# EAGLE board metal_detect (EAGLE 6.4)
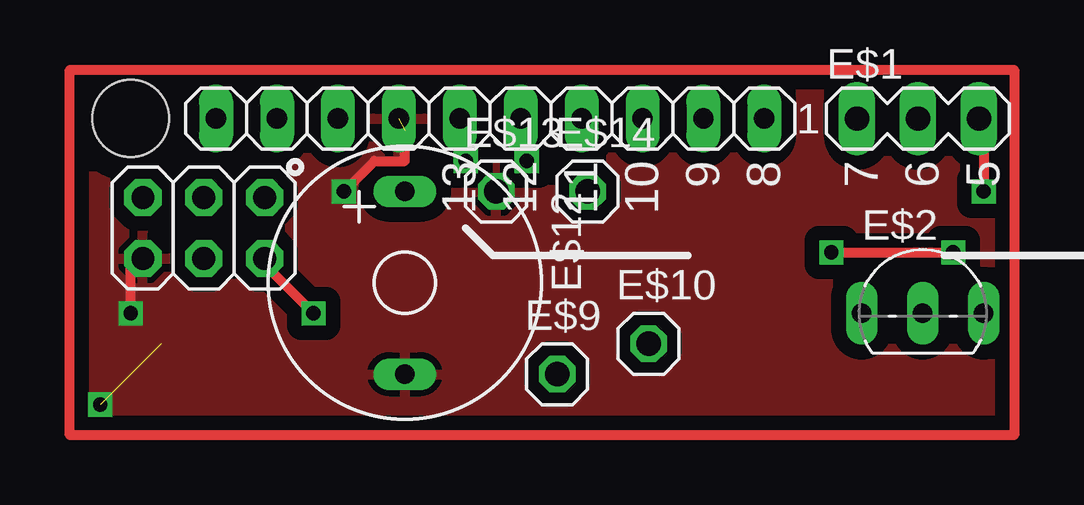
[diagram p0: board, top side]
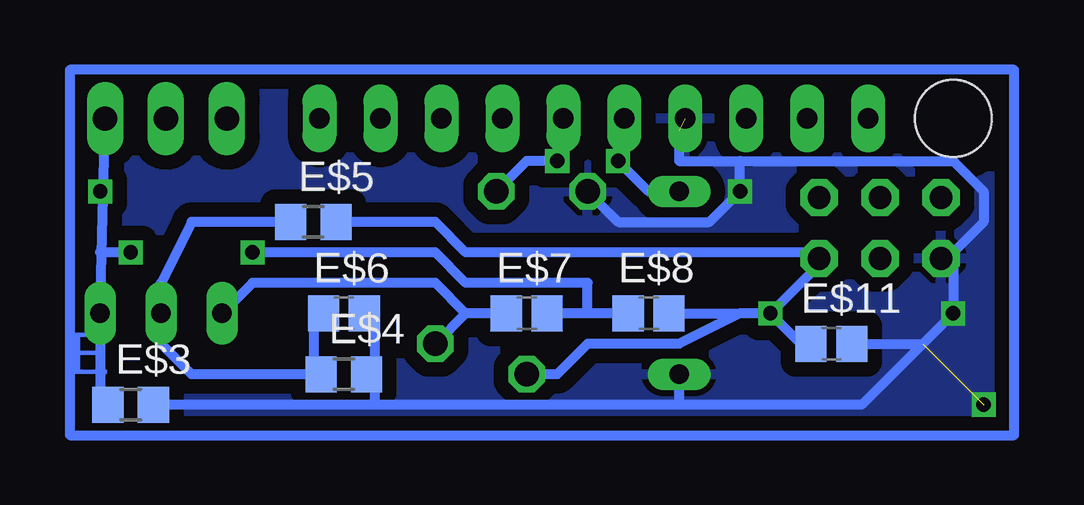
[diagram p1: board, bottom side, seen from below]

No outline drawn. Coordinates in mm, seen from the top.
Copper layers (1*16): Top 0.035mm / dielectric 1.5mm / Bottom 0.035mm
Design rules "default *": minimum track width 10mil, minimum drill 24mil, track to track 24mil, track to pad 24mil, pad to pad 24mil, via to via 24mil, smd to smd 24mil, copper to edge 40mil, drill to drill 8mil, minimum pad ring 10mil, minimum via ring 8mil, stop-mask expansion 4mil, vias tented up to drill 0mil, thermal gap 10mil
Net classes: 0 default: width 0.254 mm, clearance 0.254 mm; 2 gnd: width 0.305 mm, drill 0.559 mm, clearance 0.254 mm; 3 usbvcc: width 0.508 mm, drill 0.61 mm, clearance 0.254 mm; 4 aref: width 0.406 mm, drill 0.61 mm, clearance 0.254 mm
Holes 3.2 mm at 2.54,13.21

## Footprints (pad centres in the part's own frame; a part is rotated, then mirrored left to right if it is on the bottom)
MA03-1 = drill 1.016 long: 1 -2.54,0; 2 0,0; 3 2.54,0
TO92-BCE = drill 0.813 long: B 2.54,0; C 0,0; E -2.54,0
R0805 = smd 1.3 x 1.5: 1 -0.95,0; 2 0.95,0
C2012 = smd 1.3 x 1.5: 1 -0.85,0; 2 0.85,0
1X01 = drill 1.016 octagon: 1 0,0
BEEPER = drill 0.813 long: 1 -3.81,0; 2 3.81,0
2X03 = drill 0.95 pad 1.55 octagon: 1 -2.54,-1.27; 2 -2.54,1.27; 3 0,-1.27; 4 0,1.27; 5 2.54,-1.27; 6 2.54,1.27
1X10@1 = drill 0.85 pad 1.422 long: 1 -11.43,0; 2 -8.89,0; 3 -6.35,0; 4 -3.81,0; 5 -1.27,0; 6 1.27,0; 7 3.81,0; 8 6.35,0; 9 8.89,0; 10 11.43,0

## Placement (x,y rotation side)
E$1  [MA03-1]  35.36,13.2 0 top
E$2  [TO92-BCE]  35.56,5.08 0 top
E$3  1,2k  [R0805]  36.83,1.27 0 bottom
E$4  10k  [R0805]  27.94,2.54 0 bottom
E$5  1k  [R0805]  29.21,8.89 0 bottom
E$6  100n  [C2012]  27.94,5.08 0 bottom
E$7  22n  [C2012]  20.32,5.08 0 bottom
E$8  22n  [C2012]  15.24,5.08 0 bottom
E$9  [1X01]  20.32,2.54 0 top
E$10  [1X01]  24.13,3.81 0 top
E$11  100n  [C2012]  7.62,3.81 0 bottom
E$12  [BEEPER]  13.97,6.35 270 top
E$13  [1X01]  17.78,10.16 0 top
E$14  [1X01]  21.59,10.16 0 top
ICSP1  3x2 M  [2X03]  5.59,8.64 180 top
IOH  10x1F-H8.5  [1X10@1]  17.53,13.21 180 top

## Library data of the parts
E$1 = con-lstb
E$2 = transistor-npn
E$3-E$8 E$11 = rcl
E$9 E$10 E$13 E$14 = pinhead
E$12 = special
ICSP1 IOH = SmartPrj

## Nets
+5V [usbvcc]: ICSP1.2
AD4/SDA: IOH.9
AD5/SCL: IOH.10
AREF [aref]: IOH.8
GND [gnd]: E$12.2 E$13.1 ICSP1.6 IOH.7
IO8: IOH.1
IO9: IOH.2
MISO: IOH.5
MISO2: ICSP1.1
MOSI: IOH.4
MOSI2: ICSP1.4
RESET2: ICSP1.5
S$2: E$1.3 E$2.B
S$3: E$2.C
S$4: E$9.1
S$7: E$2.E
S$8: E$12.1
S$10: E$14.1
SCK: IOH.6
SCK2: ICSP1.3
SS: IOH.3

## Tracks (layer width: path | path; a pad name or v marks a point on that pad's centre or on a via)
GND  (via drill 0.6)  (2 unrouted)
  Top 0.406: v11.43,10.16 12.7,11.43 13.97,11.43 13.97,12.7 | v2.54,5.08 2.54,7.62
  Bottom 0.406: 26.67,1.27 35.56,1.27 | 3.81,3.81 v2.54,5.08 2.54,7.62 1.27,8.89 1.27,10.16 2.54,11.43 11.43,11.43 | 3.81,3.81 6.35,1.27 13.97,1.27 | 13.97,1.27 26.67,1.27 | 13.97,12.7 13.97,11.43 11.43,11.43 | 26.67,5.08 26.67,1.27 | 6.35,3.81 3.81,3.81 | E$12.2 13.97,1.27 | E$13.1 16.51,8.89 12.7,8.89 v11.43,10.16 11.43,11.43
  other vias: 1.27,1.27
  pour Bottom: 0,0 0,15.24 39.37,15.24 39.37,0
  pour Top: 0,0 0,15.24 39.37,15.24 39.37,0
S$1
  Bottom 0.406: 0,0 0,15.24 39.37,15.24 39.37,0 0,0
S$2
  Bottom 0.406: 38.1,1.27 E$2.B E$1.3
S$3
  Bottom 0.406: E$2.C 35.56,3.81 34.29,2.54 29.21,2.54 29.21,5.08
S$4  (via drill 0.6)
  Top 0.406: v10.16,5.08 7.62,7.62
  Bottom 0.406: 27.94,8.89 24.13,8.89 22.86,7.62 7.62,7.62 v10.16,5.08 | 13.97,5.08 11.43,5.08 | v10.16,5.08 11.43,5.08 | 8.89,3.81 v10.16,5.08 | 11.43,5.08 13.97,3.81 17.78,3.81 19.05,2.54 E$9.1
S$5
  Bottom 0.406: 30.48,8.89 34.29,8.89 35.56,6.35
S$6  (via drill 0.6)
  Top 0.406: v31.75,7.62 v36.83,7.62
  Bottom 0.406: 16.51,5.08 17.78,5.08 | 17.78,5.08 19.05,5.08 | 17.78,5.08 17.78,6.35 22.86,6.35 24.13,7.62 v31.75,7.62 | v36.83,7.62 38.1,7.62
S$7
  Bottom 0.406: 21.59,5.08 22.86,5.08 | 22.86,5.08 24.13,6.35 31.75,6.35 E$2.E | 22.86,5.08 24.13,3.81
S$8  (via drill 0.6)
  Top 0.406: v16.51,11.43 16.51,12.7
  Bottom 0.406: E$12.1 15.24,10.16 v16.51,11.43 16.51,12.7
S$9
  Top 0.406: 0,0 0,15.24 39.37,15.24 39.37,0 0,0
S$10  (via drill 0.6)
  Top 0.406: v19.05,11.43 19.05,12.7
  Bottom 0.406: 19.05,12.7 v19.05,11.43 20.32,11.43 E$14.1
S$11  (via drill 0.6)
  Top 0.406: 38.1,12.7 v38.1,10.16

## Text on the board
Bottom: E
tPlace: 13 | 12 | 11 | 10 | 9 | 8 | 7 | 6 | 5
